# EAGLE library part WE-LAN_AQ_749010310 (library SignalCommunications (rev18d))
WE-LAN AQ 10/100 Base-T SMD Transformer 1 Port Characteristics 100 % machine production High performance return loss and crosstalk Improved solderability through half vias Reduced height (4 mm) Compatible to standard products Applications Compatible to industrial ethernet systems like EtherCAT or Profinet IoT applications Hubs, routers, switches, IPcameras Company networks Details see: http://katalog.we-online.de/en/pbs/WE-LANAQ Created by Yingchun Shan 2017 (C) Wurth Elektronik
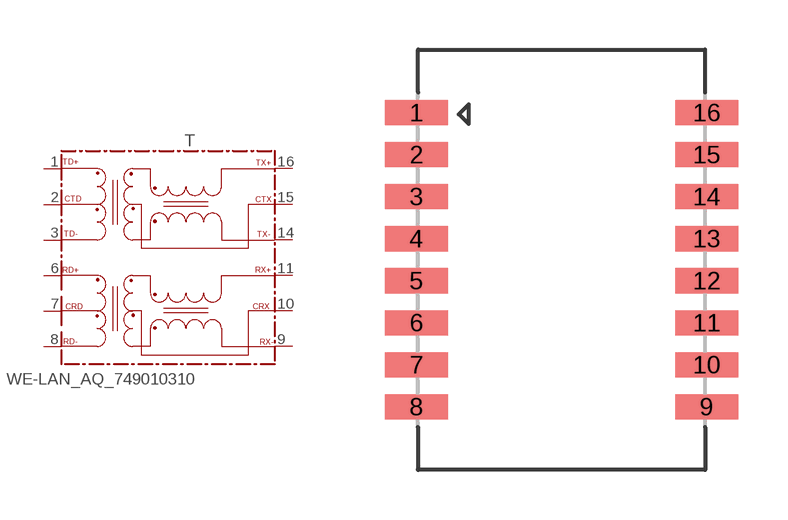
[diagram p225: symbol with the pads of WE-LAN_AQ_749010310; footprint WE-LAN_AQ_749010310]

Designator prefix T

## WE-LAN_AQ_749010310  [WE-LAN_AQ_749010310]
1  TD+
2  CTD
3  TD-
6  RD+
7  CRD
8  RD-
9  RX-
10  CRX
11  RX+
14  TX-
15  CTX
16  TX+

## Footprint WE-LAN_AQ_749010310 (pad centres in mm)
smd 1.9 x 0.76: 1 -4.385,4.445; 2 -4.385,3.175; 3 -4.385,1.905; 4 -4.385,0.635; 5 -4.385,-0.635; 6 -4.385,-1.905; 7 -4.385,-3.175; 8 -4.385,-4.445; 9 4.385,-4.445; 10 4.385,-3.175; 11 4.385,-1.905; 12 4.385,-0.635; 13 4.385,0.635; 14 4.385,1.905; 15 4.385,3.175; 16 4.385,4.445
